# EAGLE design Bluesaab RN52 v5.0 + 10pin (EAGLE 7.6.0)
Removed DFU switch! D3 CANNOT be a Schottky diode; needs to be a signal diode. Might as well make all diodes the same... Added 2 bypass caps to RN52 power line. Switched to SN65HVD234 for higher temp (also has Enable pin which needs pulled high). Added 10 pin connector for the daughter board Amplifier. - OTHERWISE, THE LEFT 4 COLUMNS NEED JUMPERED.
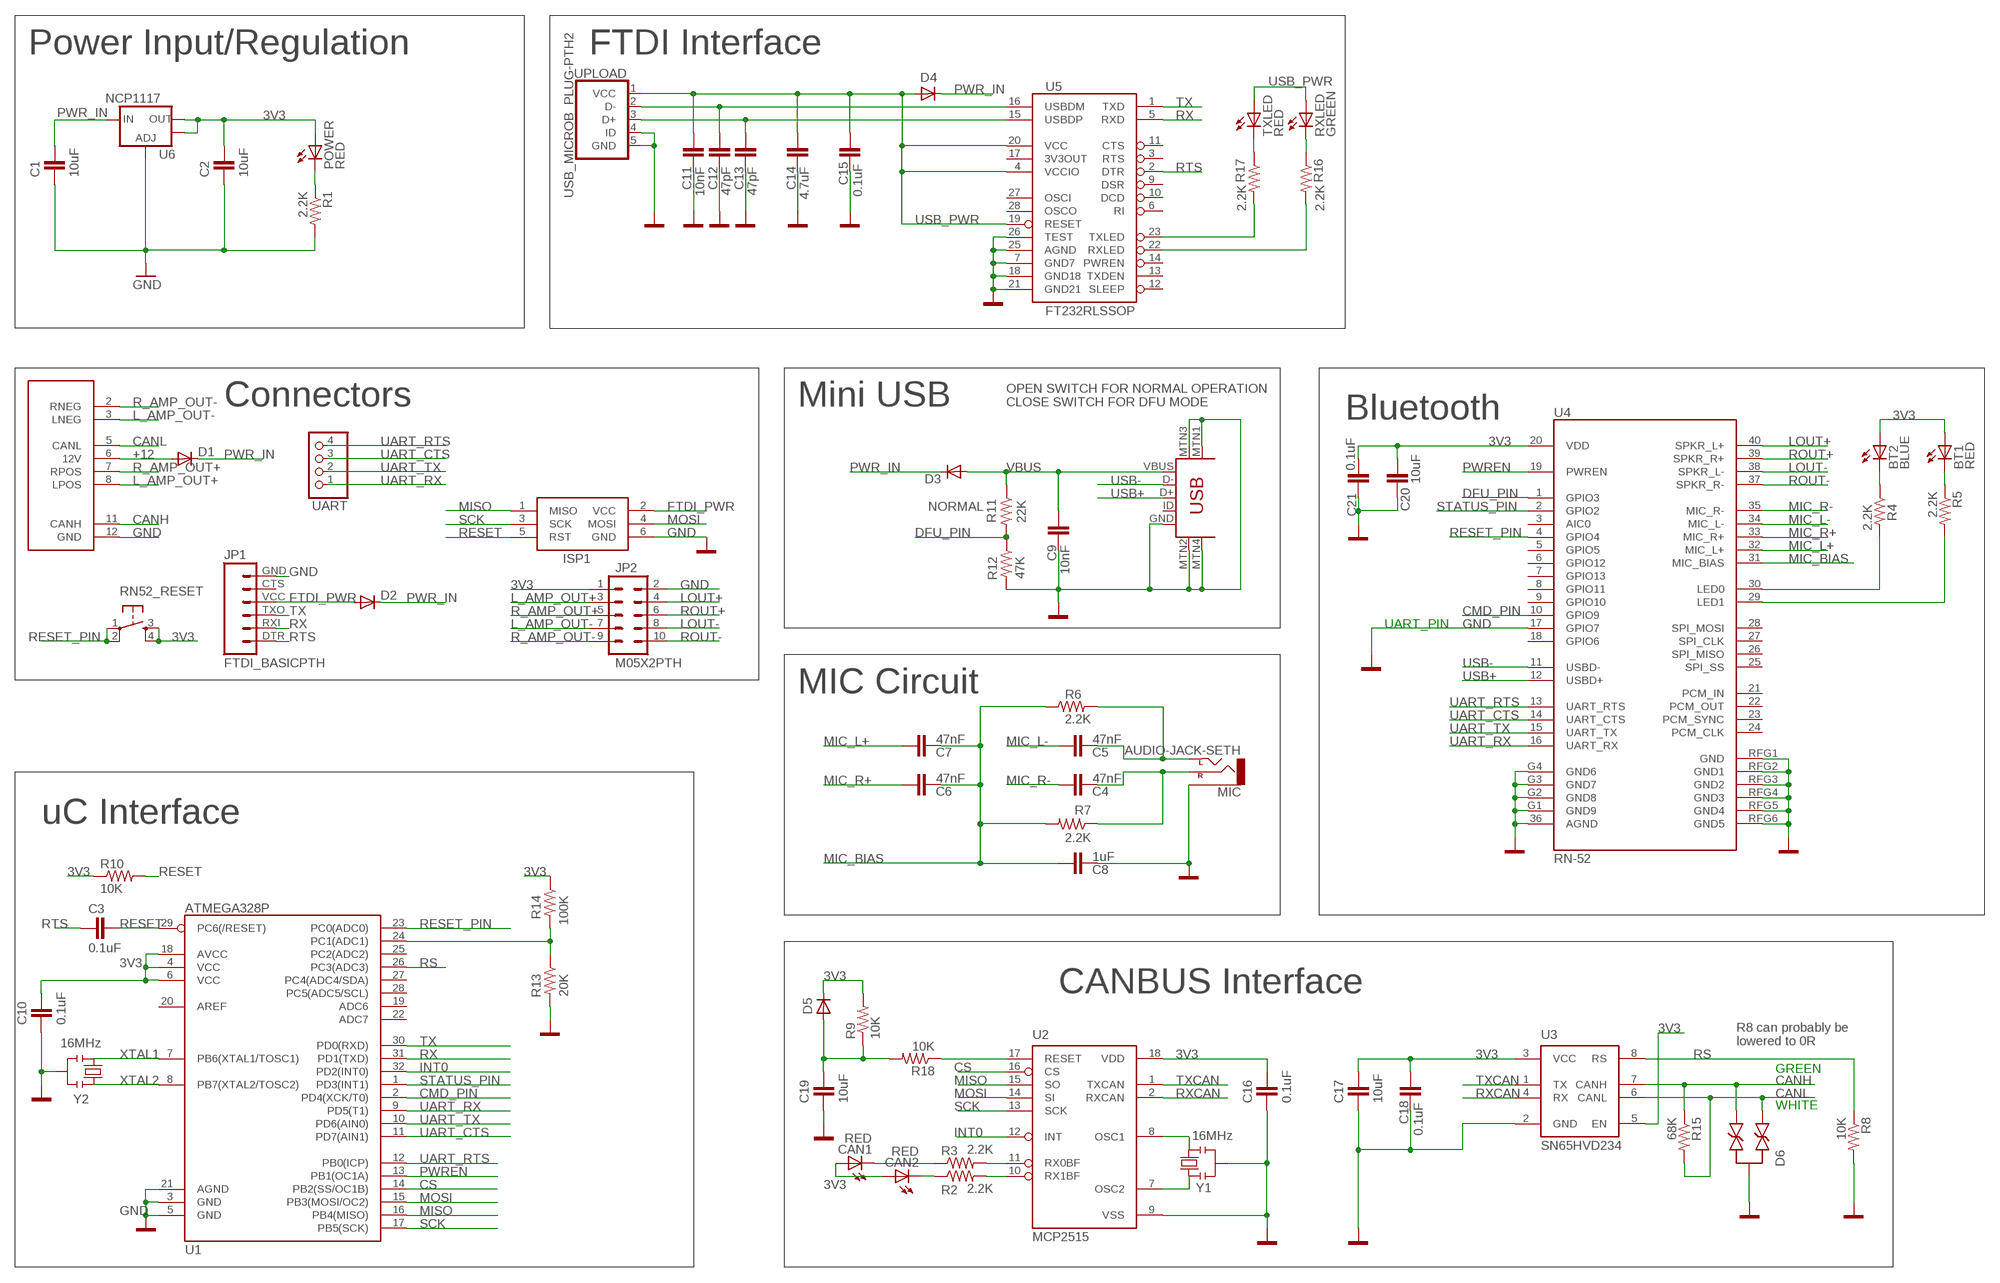
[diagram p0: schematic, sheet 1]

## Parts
BT1  RED  LEDSML1206  [SML1206]
BT2  BLUE  LEDSML1206  [SML1206]
C1  10uF  C-EUC0805K  [C0805K]
C2  10uF  C-EUC0805K  [C0805K]
C3  0.1uF  C-EUC0805K  [C0805K]
C4  47nF  C-EUC0805K  [C0805K]
C5  47nF  C-EUC0805K  [C0805K]
C6  47nF  C-EUC0805K  [C0805K]
C7  47nF  C-EUC0805K  [C0805K]
C8  1uF  C-EUC0805K  [C0805K]
C9  10nF  C-EUC0805K  [C0805K]
C10  0.1uF  C-EUC0805K  [C0805K]
C11  10nF  C-EUC0805K  [C0805K]
C12  47pF  C-EUC0805K  [C0805K]
C13  47pF  C-EUC0805K  [C0805K]
C14  4.7uF  C-EUC0805K  [C0805K]
C15  0.1uF  C-EUC0805K  [C0805K]
C16  0.1uF  C-EUC0805K  [C0805K]
C17  10uF  C-EUC0805K  [C0805K]
C18  0.1uF  C-EUC0805K  [C0805K]
C19  10uF  C-EUC0805K  [C0805K]
C20  10uF  C-EUC0805K  [C0805K]
C21  0.1uF  C-EUC0805K  [C0805K]
CAN1  RED  LEDSML1206  [SML1206]
CAN2  RED  LEDSML1206  [SML1206]
D1  DIODE-SCHOTTKY_  DIODE-SOD123  [SOD123]
D2  DIODE-SCHOTTKY_  DIODE-SOD123  [SOD123]
D3  DIODE-SCHOTTKY_  DIODE-SOD123  [SOD123]
D4  DIODE-SCHOTTKY_  DIODE-SOD123  [SOD123]
D5  DIODE-SCHOTTKY_  DIODE-SOD123  [SOD123]
D6  DIODE-ARRAY  [SOT23]
ISP1  AVRISP-6  [AVRISP]
JP1  FTDI_BASICPTH  [FTDI_BASIC]
JP2  M05X2PTH  [AVR_ICSP]
MIC  AUDIO-JACK-SETH  [AUDIO-JACK-3.5MM-SMD-SETH]
POWER  RED  LEDSML1206  [SML1206]
R1  2.2K  R-US_R0805  [R0805]
R2  2.2K  R-US_R0805  [R0805]
R3  2.2K  R-US_R0805  [R0805]
R4  2.2K  R-US_R0805  [R0805]
R5  2.2K  R-US_R0805  [R0805]
R6  2.2K  R-US_R0805  [R0805]
R7  2.2K  R-US_R0805  [R0805]
R8  10K  R-US_R0805  [R0805]
R9  10K  R-US_R0805  [R0805]
R10  10K  R-US_R0805  [R0805]
R11  22K  R-US_R0805  [R0805]
R12  47K  R-US_R0805  [R0805]
R13  20K  R-US_R0805  [R0805]
R14  100K  R-US_R0805  [R0805]
R15  68K  R-US_R0805  [R0805]
R16  2.2K  R-US_R0805  [R0805]
R17  2.2K  R-US_R0805  [R0805]
R18  10K  R-US_R0805  [R0805]
RN52_FIRMWARE  USB-MINIB-5PIN  [USB-MINIB]
RN52_RESET  TAC_SWITCH  [TACTILE_SWITCH_SMD_6MM]
RXLED  GREEN  LEDSML1206  [SML1206]
TXLED  RED  LEDSML1206  [SML1206]
U1  ATMEGA328P  ATMEGA328_SMT  [TQFP32-08]
U2  MCP2515  [SO18L]
U3  SN65HVD234  [SO8]
U4  RN-52  BLUETOOTH-RN-52  [RN-52]
U5  FT232RLSSOP  [SSOP28DB]
U6  NCP1117  V_REG_LM1117SOT223  [SOT223]
U$5  827229-1  [827229-1]
UART  PINHD-1X4  [1X04]
UPLOAD  USB_MICROB_PLUG-PTH2  [MICRO-B-TH]
Y1  16MHz  RESONATORSMD  [RESONATOR-SMD]
Y2  16MHz  RESONATORSMD  [RESONATOR-SMD]

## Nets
3V3: BT1.A BT2.A C2.2 C10.2 C16.2 C17.2 C18.1 C20.1 C21.2 CAN1.A CAN2.A D5.C JP2.1 POWER.A R9.2 R10.1 R14.1 RN52_RESET.3 RN52_RESET.4 U1.4(VCC) U1.6(VCC) U1.18(AVCC) U2.18(VDD) U3.3(VCC) U3.5(EN) U4.20(VDD) U6.2(OUT) U6.4(OUT)
+12 [12v]: D1.A U$5.6(12V)
CANH: D6.2 R15.1 U3.7(CANH) U$5.11(CANH)
CANL: D6.1 R15.2 U3.6(CANL) U$5.5(CANL)
CMD_PIN: U1.2(PD4(XCK/T0)) U4.10(GPIO9)
CS: U1.14(PB2(SS/OC1B)) U2.16(CS)
DFU_PIN: R11.2 R12.1 U4.1(GPIO3)
FTDI_PWR: D2.A ISP1.2(VCC) JP1.VCC
GND: C1.1 C2.1 C8.1 C9.1 C10.1 C11.1 C12.1 C13.1 C14.1 C15.2 C16.1 C17.1 C18.2 C19.1 C20.2 C21.1 D6.3 ISP1.6(GND) JP1.GND JP2.2 MIC.SLEEVE R1.2 R8.2 R12.2 R13.2 RN52_FIRMWARE.GND RN52_FIRMWARE.MTN1(MTN2) RN52_FIRMWARE.MTN2(MTN3) RN52_FIRMWARE.MTN3(MTN1) RN52_FIRMWARE.MTN4 U1.3(GND) U1.5(GND) U1.21(AGND) U2.9(VSS) U3.2(GND) U4.17(GPIO7) U4.36(AGND) U4.G1(GND9) U4.G2(GND8) U4.G3(GND7) U4.G4(GND6) U4.RFG1(GND) U4.RFG2(GND1) U4.RFG3(GND2) U4.RFG4(GND3) U4.RFG5(GND4) U4.RFG6(GND5) U5.7(GND7) U5.18(GND18) U5.21(GND21) U5.25(AGND) U5.26(TEST) U6.1(ADJ) U$5.12(GND) UPLOAD.4(ID) UPLOAD.5(GND) Y1.2 Y2.2
INT0: U1.32(PD2(INT0)) U2.12(INT)
L_AMP_OUT+: JP2.3 U$5.8(LPOS)
L_AMP_OUT-: JP2.7 U$5.3(LNEG)
LOUT+: JP2.4 U4.40(SPKR_L+)
LOUT-: JP2.8 U4.38(SPKR_L-)
MIC_BIAS: C6.1 C7.1 C8.2 R6.1 R7.2 U4.31(MIC_BIAS)
MIC_L+: C7.2 U4.32(MIC_L+)
MIC_L-: C5.1 U4.34(MIC_L-)
MIC_R+: C6.2 U4.33(MIC_R+)
MIC_R-: C4.1 U4.35(MIC_R-)
MISO: ISP1.1(MISO) U1.16(PB4(MISO)) U2.15(SO)
MOSI: ISP1.4(MOSI) U1.15(PB3(MOSI/OC2)) U2.14(SI)
N$1: R16.2 U5.22(RXLED)
N$4: U2.8(OSC1) Y1.3
N$5: U2.7(OSC2) Y1.1
N$6: BT2.C R4.1
N$7: BT1.C R5.1
N$8: R18.1 U2.17(RESET)
N$9: R13.1 R14.2 U1.24(PC1(ADC1))
N$10: R17.2 U5.23(TXLED)
N$12: R16.1 RXLED.C
N$13: CAN1.C R3.1
N$15: R17.1 TXLED.C
N$16: CAN2.C R2.1
N$17: POWER.C R1.1
N$18: R3.2 U2.11(RX0BF)
N$23: C4.2 MIC.RING(RIGHT) R7.1
N$25: C5.2 MIC.TIP(LEFT) R6.2
N$28: R5.2 U4.29(LED1)
N$29: R4.2 U4.30(LED0)
N$31: R2.2 U2.10(RX1BF)
N$35: C19.2 D5.A R9.1 R18.2
PWR_IN [12v]: C1.2 D1.C D2.C D3.C D4.C U6.3(IN)
PWREN: U1.13(PB1(OC1A)) U4.19(PWREN)
R_AMP_OUT+: JP2.5 U$5.7(RPOS)
R_AMP_OUT-: JP2.9 U$5.2(RNEG)
RESET: C3.2 ISP1.5(RST) R10.2 U1.29(PC6(/RESET))
RESET_PIN: RN52_RESET.1 RN52_RESET.2 U1.23(PC0(ADC0)) U4.4(GPIO4)
ROUT+: JP2.6 U4.39(SPKR_R+)
ROUT-: JP2.10 U4.37(SPKR_R-)
RS: R8.1 U1.26(PC3(ADC3)) U3.8(RS)
RTS: C3.1 JP1.DTR U5.2(DTR)
RX: JP1.RXI U1.31(PD1(TXD)) U5.5(RXD)
RXCAN: U2.2(RXCAN) U3.4(RX)
SCK: ISP1.3(SCK) U1.17(PB5(SCK)) U2.13(SCK)
STATUS_PIN: U1.1(PD3(INT1)) U4.2(GPIO2)
TX: JP1.TXO U1.30(PD0(RXD)) U5.1(TXD)
TXCAN: U2.1(TXCAN) U3.1(TX)
UART_CTS: U1.11(PD7(AIN1)) U4.14(UART_CTS) UART.3
UART_RTS: U1.12(PB0(ICP)) U4.13(UART_RTS) UART.4
UART_RX: U1.9(PD5(T1)) U4.16(UART_RX) UART.1
UART_TX: U1.10(PD6(AIN0)) U4.15(UART_TX) UART.2
USB+: RN52_FIRMWARE.D+ U4.12(USBD+)
USB-: RN52_FIRMWARE.D- U4.11(USBD-)
USB_PWR: C11.2 C14.2 C15.1 D4.A RXLED.A TXLED.A U5.4(VCCIO) U5.19(RESET) U5.20(VCC) UPLOAD.1(VCC)
USBDM: C12.2 U5.16(USBDM) UPLOAD.2(D-)
USBDP: C13.2 U5.15(USBDP) UPLOAD.3(D+)
VBUS: C9.2 D3.A R11.1 RN52_FIRMWARE.VBUS
XTAL1: U1.7(PB6(XTAL1/TOSC1)) Y2.1
XTAL2: U1.8(PB7(XTAL2/TOSC2)) Y2.3
Unconnected: JP1.CTS RN52_FIRMWARE.ID U1.19(ADC6) U1.20(AREF) U1.22(ADC7) U1.25(PC2(ADC2)) U1.27(PC4(ADC4/SDA)) U1.28(PC5(ADC5/SCL)) U4.3(AIC0) U4.5(GPIO5) U4.6(GPIO12) U4.7(GPIO13) U4.8(GPIO11) U4.9(GPIO10) U4.18(GPIO6) U4.21(PCM_IN) U4.22(PCM_OUT) U4.23(PCM_SYNC) U4.24(PCM_CLK) U4.25(SPI_SS) U4.26(SPI_MISO) U4.27(SPI_CLK) U4.28(SPI_MOSI) U5.3(RTS) U5.6(RI) U5.9(DSR) U5.10(DCD) U5.11(CTS) U5.12(SLEEP) U5.13(TXDEN) U5.14(PWREN) U5.17(3V3OUT) U5.27(OSCI) U5.28(OSCO)

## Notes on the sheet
- Power Input/Regulation | FTDI Interface
- Connectors | Mini USB
- OPEN SWITCH FOR NORMAL OPERATION
  CLOSE SWITCH FOR DFU MODE
- Bluetooth
- NORMAL
- UART_PIN
- MIC Circuit
- uC Interface
- CANBUS Interface
- R8 can probably be
  lowered to 0R
- GREEN
- WHITE

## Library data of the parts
BT1 BT2 CAN1 CAN2 POWER RXLED TXLED = led:LED: LED
C1-C21 = rcl:C-EU: CAPACITOR, European symbol
D1-D5 = diode_seth:DIODE-: DIODE
D6 = SparkFun-seth:DIODE-ARRAY: NUP2105L, TVS Diode Array
ISP1 = adafruit:AVRISP: AVR ISP HEADER Standard 6 pin header for AVR programming
JP1 = SparkFun-seth:FTDI_BASIC: FTDI Basic: 3.3V and 5V
JP2 = SparkFun-Connectors:M05X2: Header 5x2 Standard 10-pin dual row 0.1" header. Commonly used with AVR-ISP. Use with Spark Fun Electronics SKU: PRT-00778
MIC = SparkFun-Connectors:AUDIO-JACK-SETH
R1-R18 = rcl:R-US_: RESISTOR, American symbol
RN52_FIRMWARE = SparkFun-Connectors:USB-MINIB: Mini-USB "B" connector with 5th pin broken out. Created new symbol breaking out 5th "ID" pin in mini/micro USB connector spec. See: http://en.wikipedia.org/wiki/Mini_usb#Cables. Uses same footprint as 4-pin symbol. Also added pins to connect to mounting / shield pads if required (probably not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
RN52_RESET = SparkFun-seth:TAC_SWITCH: Momentary Switch Button commonly used for reset or general input. Spark Fun Electronics SKU : COM-00097
U1 = SparkFun-DigitalIC:ATMEGA328_SMT: 32-Pin Atmega328 part Commonly used on Arduino compatible boards Available in QFP and QFN packages TQFP is IC-09069 QFN is non-stock; PROD_ID: IC-09069
U2 = mcp2515-seth:MCP2515
U3 = ti-can-seth:SN65HVD234
U4 = SparkFun-RF:BLUETOOTH-RN-52
U5 = SparkFun-DigitalIC:FT232RL: USB UART FT232RL 4th Generation USB UART (USB <-> Serial) Controller. Spark Fun Electronics SKU : COM-00650 Production SKU IC-00870; PROD_ID: IC-00870
U6 = SparkFun:V_REG_LM1117: Voltage Regulator LM1117 Standard adjustable voltage regulator but in SMD form. Spark Fun Electronics SKU : COM-00595
U$5 = 827229-1:827229-1
UART = pinhead:PINHD-1X4: PIN HEADER
UPLOAD = SparkFun-Connectors-seth:USB_MICROB_PLUG: USB Micro-B Plug Comes in a variety of packages. Check out Hirose's ZX-x0 line: http://www.hirose.co.jp/cataloge_hp/e24200011.pdf
Y1 Y2 = SparkFun-seth:RESONATOR: Resonator Small SMD resonator. This is the itty bitty 10/20MHz resonators with built in caps. CSTCE10M0G55 and CSTCE20M0V53. Footprint has been reviewed closely but hasn't been tested yet.

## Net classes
0 default: width 0.254 mm
1 12v: width 0.5 mm

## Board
New PCB design, based on v4.4, NOW with 0805 resistors and caps. Adjusted layout to account for smaller parts.
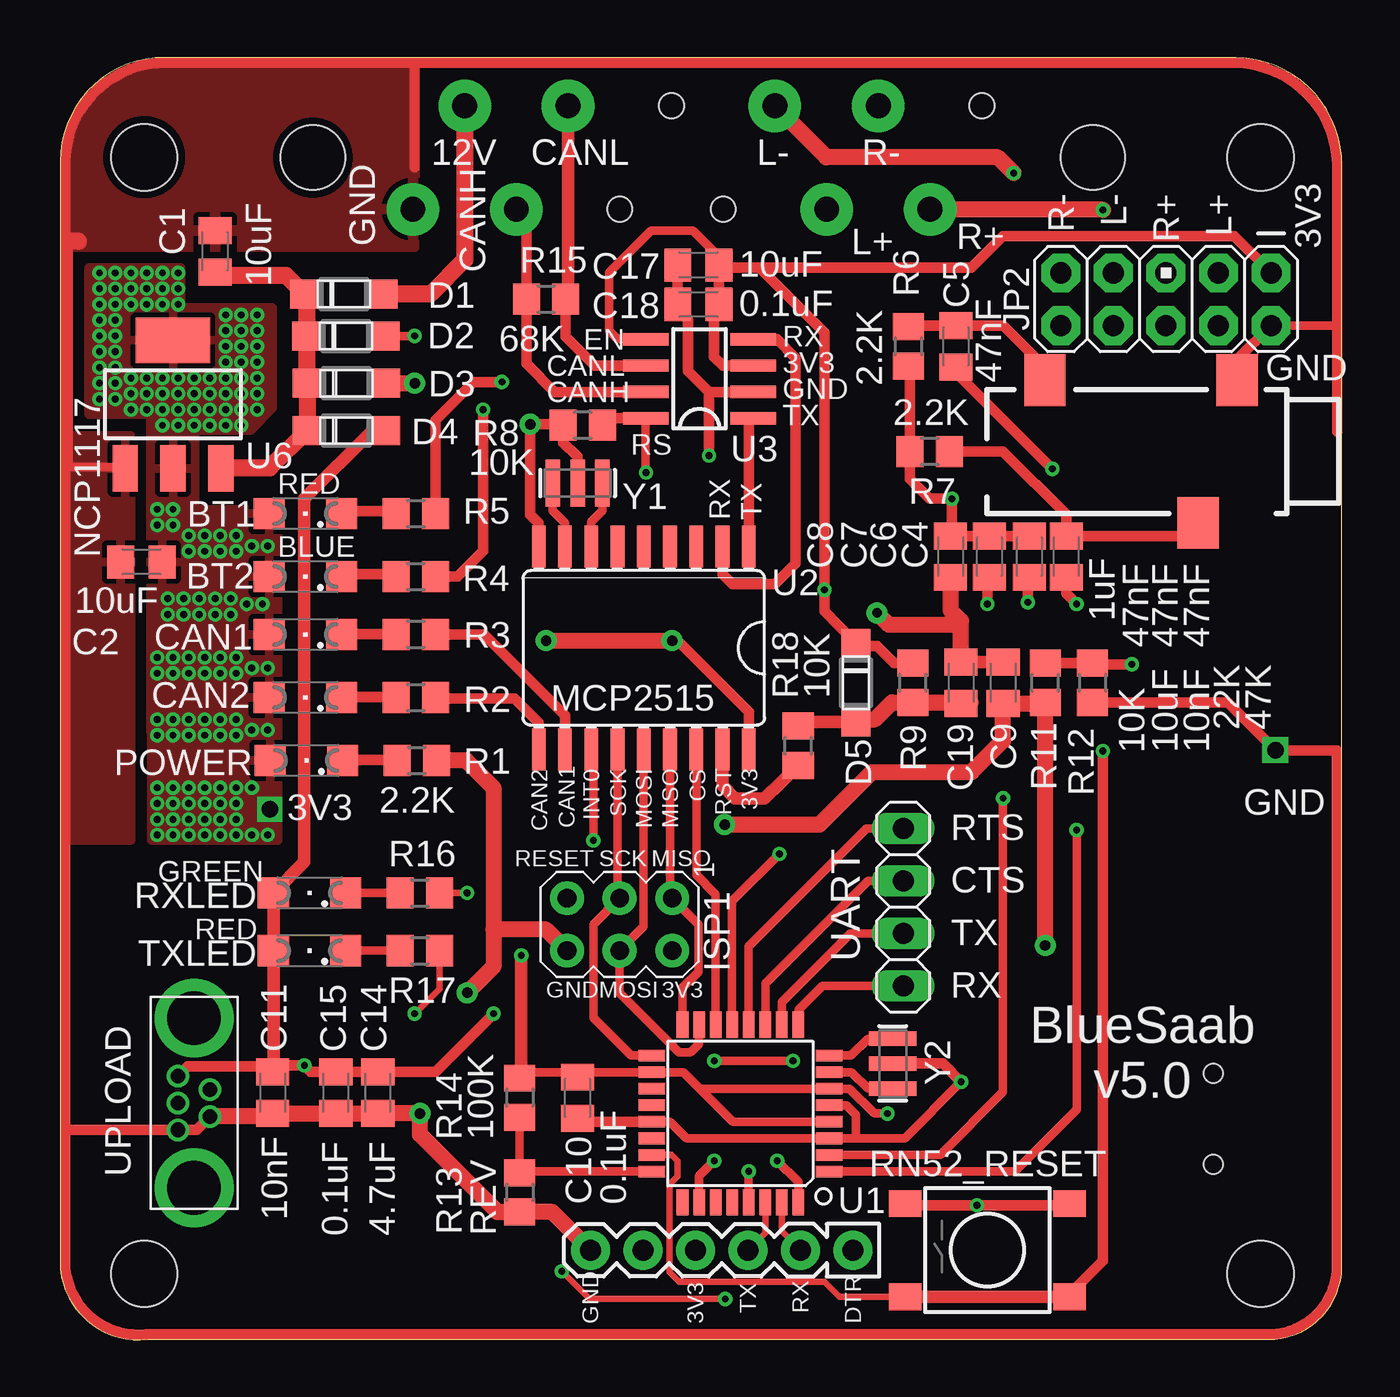
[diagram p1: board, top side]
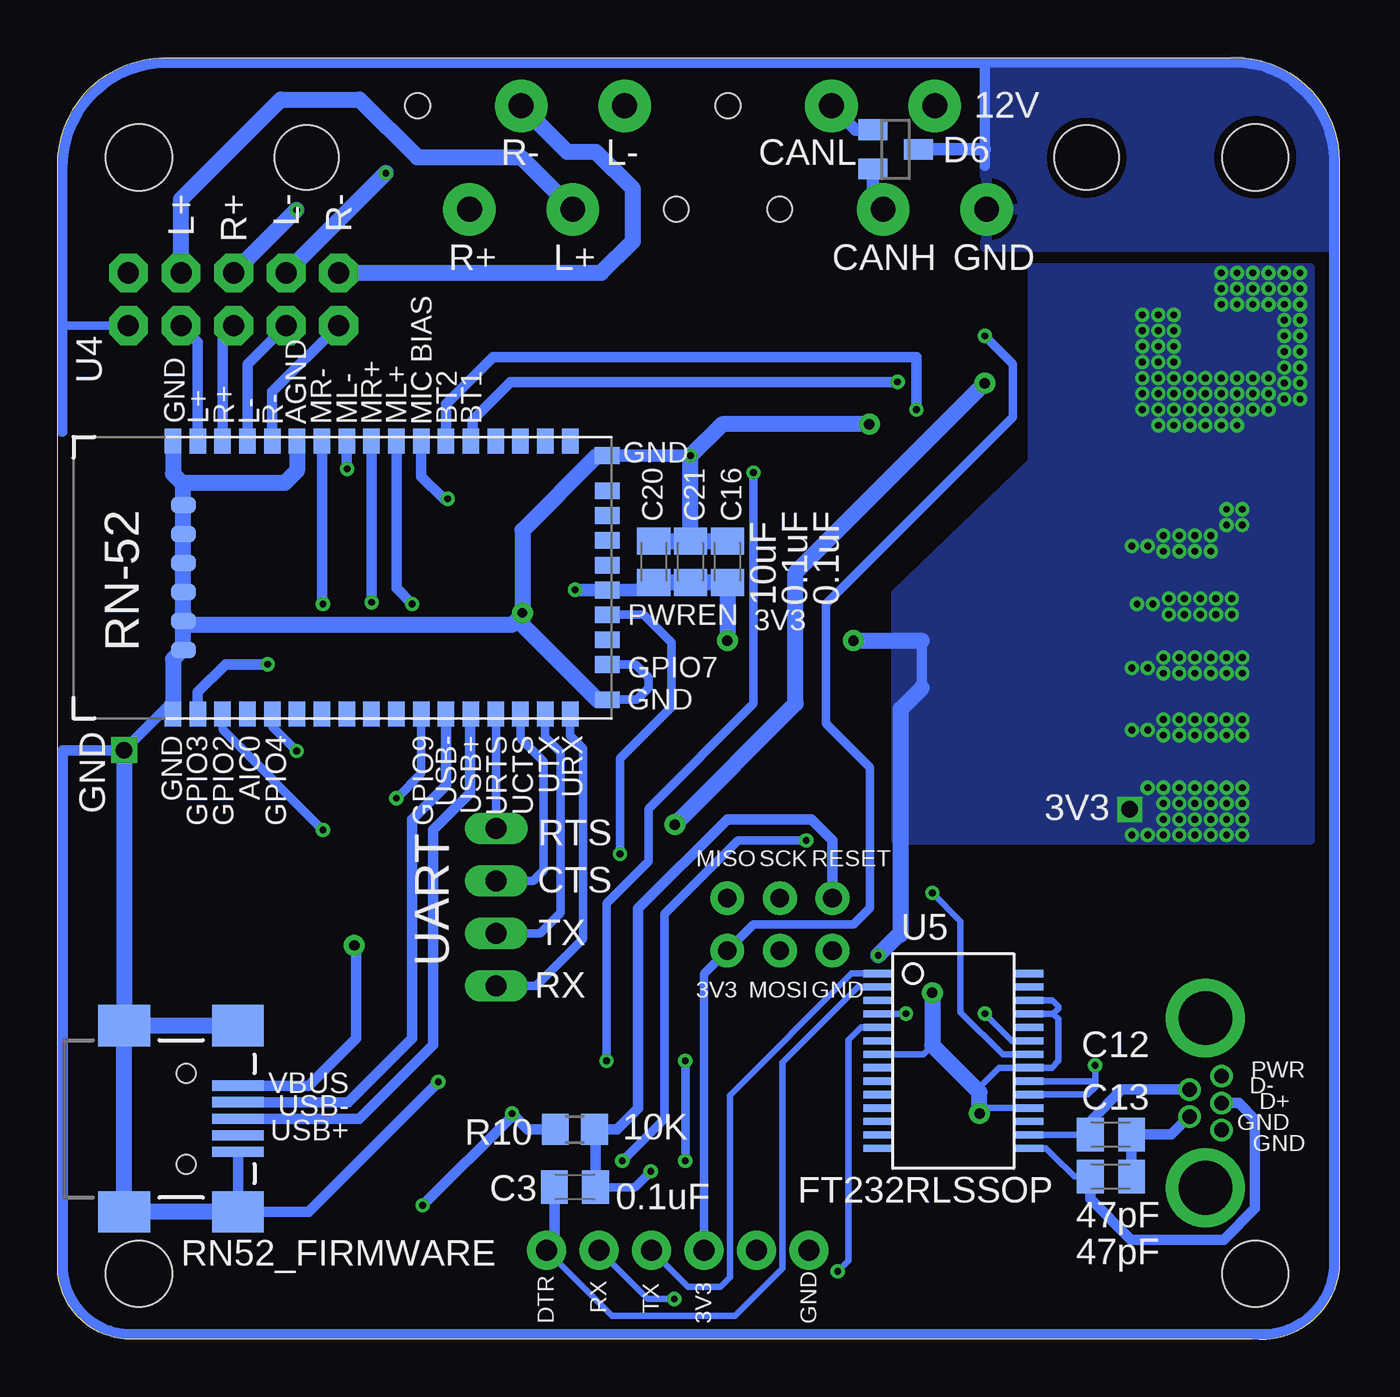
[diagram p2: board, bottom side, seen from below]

Size 61.98 x 62 mm. Coordinates in mm from the lower left corner, seen from the top.
Outline: 56.86,62 5.06,62 arc90 0,56.97 0,3.42 arc90 4.24,0.02 58.4,0.02 arc90 61.98,3.53 61.98,56.71 arc90 56.86,62
Copper layers (1*16): Top 0.0356mm / dielectric 1.5011mm / Bottom 0.0356mm
Design rules "OSHPark": minimum track width 6mil, minimum drill 13mil, track to track 6mil, track to pad 6mil, pad to pad 6mil, via to via 6mil, smd to smd 6mil, copper to edge 15mil, drill to drill 6mil, minimum pad ring 7mil, minimum via ring 7mil, stop-mask expansion 4mil, vias tented up to drill 0mil, thermal gap 10mil
Holes 3.2 mm at 4.06,57.17 58.04,57.17 58.04,3.2 4.06,3.2

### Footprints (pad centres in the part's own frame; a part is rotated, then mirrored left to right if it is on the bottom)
SML1206 = smd 1.5 x 1.5: A 1.75,0; C -1.75,0
C0805K = smd 1.3 x 1.6: 1 -1,0; 2 1,0
SOD123 = smd 1.4 x 1.4: A 1.9,0; C -1.9,0
SOT23 = smd 1 x 1.4: 1 -0.95,-1.1; 2 0.95,-1.1; 3 0,1.1
AVRISP = drill 0.9 pad 1.626: 1 -1.27,2.54; 2 1.27,2.54; 3 -1.27,0; 4 1.27,0; 5 -1.27,-2.54; 6 1.27,-2.54
FTDI_BASIC = drill 1.016 pad 1.88: CTS 10.16,0; DTR 0,0; GND 12.7,0; RXI 2.54,0; TXO 5.08,0; VCC 7.62,0
AVR_ICSP = drill 1.016 pad 1.88 octagon: 1 -1.27,5.08; 2 1.27,5.08; 3 -1.27,2.54; 4 1.27,2.54; 5 -1.27,0; 6 1.27,0; 7 -1.27,-2.54; 8 1.27,-2.54; 9 -1.27,-5.08; 10 1.27,-5.08
AUDIO-JACK-3.5MM-SMD-SETH = smd 2 x 2.5: RING 4.3,3.45; SLEEVE 2.4,-3.45; TIP 11.7,-3.45
R0805 = smd 1.3 x 1.5: 1 -0.95,0; 2 0.95,0
USB-MINIB = smd 2.5 x 0.5: D+ 2.5,0; D- 2.5,0.8; GND 2.5,-1.6; ID 2.5,-0.8; VBUS 2.5,1.6 | smd 2.5 x 2: MTN1 -3,4.5; MTN2 2.5,4.5; MTN3 -3,-4.5; MTN4 2.5,-4.5 | hole 0.9: 0,2.2; 0,-2.2
TACTILE_SWITCH_SMD_6MM = smd 1.55 x 1.3: 1 -3.975,2.25; 2 3.975,2.25; 3 -3.975,-2.25; 4 3.975,-2.25
TQFP32-08 = smd 1.27 x 0.559: 1 -4.293,2.8; 2 -4.293,2; 3 -4.293,1.2; 4 -4.293,0.4; 5 -4.293,-0.4; 6 -4.293,-1.2; 7 -4.293,-2; 8 -4.293,-2.8; 17 4.293,-2.8; 18 4.293,-2; 19 4.293,-1.2; 20 4.293,-0.4; 21 4.293,0.4; 22 4.293,1.2; 23 4.293,2; 24 4.293,2.8 | smd 0.559 x 1.27: 9 -2.8,-4.293; 10 -2,-4.293; 11 -1.2,-4.293; 12 -0.4,-4.293; 13 0.4,-4.293; 14 1.2,-4.293; 15 2,-4.293; 16 2.8,-4.293; 25 2.8,4.293; 26 2,4.293; 27 1.2,4.293; 28 0.4,4.293; 29 -0.4,4.293; 30 -1.2,4.293; 31 -2,4.293; 32 -2.8,4.293
SO18L = smd 0.66 x 2.032: 1 -5.08,-4.902; 2 -3.81,-4.902; 3 -2.54,-4.902; 4 -1.27,-4.902; 5 0,-4.902; 6 1.27,-4.902; 7 2.54,-4.902; 8 3.81,-4.902; 9 5.08,-4.902; 10 5.08,4.902; 11 3.81,4.902; 12 2.54,4.902; 13 1.27,4.902; 14 0,4.902; 15 -1.27,4.902; 16 -2.54,4.902; 17 -3.81,4.902; 18 -5.08,4.902
SO8 = smd 0.6 x 2.2: 1 -1.905,-2.6; 2 -0.635,-2.6; 3 0.635,-2.6; 4 1.905,-2.6; 5 1.905,2.6; 6 0.635,2.6; 7 -0.635,2.6; 8 -1.905,2.6
RN-52 = smd 1.2 x 0.8: 1 -6.6,8.33; 2 -6.6,7.13; 3 -6.6,5.93; 4 -6.6,4.73; 5 -6.6,3.53; 6 -6.6,2.33; 7 -6.6,1.13; 8 -6.6,-0.07; 9 -6.6,-1.27; 10 -6.6,-2.47; 11 -6.6,-3.67; 12 -6.6,-4.87; 13 -6.6,-6.07; 14 -6.6,-7.27; 15 -6.6,-8.47; 16 -6.6,-9.67; 25 6.6,-9.67; 26 6.6,-8.47; 27 6.6,-7.27; 28 6.6,-6.07; 29 6.6,-4.87; 30 6.6,-3.67; 31 6.6,-2.47; 32 6.6,-1.27; 33 6.6,-0.07; 34 6.6,1.13; 35 6.6,2.33; 36 6.6,3.53; 37 6.6,4.73; 38 6.6,5.93; 39 6.6,7.13; 40 6.6,8.33; G1 -6.6,9.53; G4 6.6,9.53 | smd 0.8 x 1.2: 17 -4.2,-11.47; 18 -3,-11.47; 19 -1.8,-11.47; 20 -0.6,-11.47; 21 0.6,-11.47; 22 1.8,-11.47; 23 3,-11.47; 24 4.2,-11.47; G2 -5.9,-11.47; G3 5.9,-11.46; RFG1 -3.5,9.03; RFG2 -2.1,9.03; RFG3 -0.7,9.03; RFG4 0.7,9.03; RFG5 2.1,9.03; RFG6 3.5,9.03
SSOP28DB = smd 0.348 x 1.397: 1 -4.225,-3.656; 2 -3.575,-3.656; 3 -2.925,-3.656; 4 -2.275,-3.656; 5 -1.625,-3.656; 6 -0.975,-3.656; 7 -0.325,-3.656; 8 0.325,-3.656; 9 0.975,-3.656; 10 1.625,-3.656; 11 2.275,-3.656; 12 2.925,-3.656; 13 3.575,-3.656; 14 4.225,-3.656; 15 4.225,3.656; 16 3.575,3.656; 17 2.925,3.656; 18 2.275,3.656; 19 1.625,3.656; 20 0.975,3.656; 21 0.325,3.656; 22 -0.325,3.656; 23 -0.975,3.656; 24 -1.625,3.656; 25 -2.275,3.656; 26 -2.925,3.656; 27 -3.575,3.656; 28 -4.225,3.656
SOT223 = smd 1.219 x 2.235: 1 -2.311,-3.099; 2 0,-3.099; 3 2.311,-3.099 | smd 3.6 x 2.2: 4 0,3.099
827229-1 = drill 1.2 pad 2.54: 2 2.96,-9.495; 3 2.96,-4.495; 5 2.96,5.505; 6 2.96,10.505; 7 -2.04,-11.995; 8 -2.04,-6.995; 11 -2.04,8.005; 12 -2.04,13.005 | hole 3.1: 0.46,17.84; 0.46,-19.86 | hole 1.2: -2.04,3.005; 2.96,-14.495; -2.04,-1.995; 2.96,0.505
1X04 = drill 1.016 long: 1 -3.81,0; 2 -1.27,0; 3 1.27,0; 4 3.81,0
MICRO-B-TH = drill 0.711 pad 1.092: 1 -1.3,-0.775; 2 -0.65,0.775; 3 0,-0.775; 4 0.65,0.775; 5 1.3,-0.775 | drill 2.591 pad 3.81: P$1 -4.1,0; P$2 4.1,0
RESONATOR-SMD = smd 0.7 x 2.286: 1 -1.2,0; 2 0,0; 3 1.2,0

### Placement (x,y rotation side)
BT1  11.86,39.95 180 top
BT2  11.86,36.9 180 top
C1  7.49,52.63 270 top
C2  3.94,37.61 0 top
C3  36.96,7.39 0 bottom
C4  48.64,37.87 90 top
C5  43.31,48.03 90 top
C6  46.86,37.87 270 top
C7  44.93,37.87 270 top
C8  43.05,37.87 90 top
C9  45.59,31.77 270 top
C10  25.02,11.71 90 top
C11  10.29,11.96 90 top
C12  11.05,9.93 180 bottom
C13  11.05,7.9 180 bottom
C14  15.37,11.96 90 top
C15  13.33,11.96 270 top
C16  29.59,37.61 270 bottom
C17  30.86,51.97 0 top
C18  30.86,50.06 180 top
C19  43.56,31.77 270 top
C20  33.15,37.61 90 bottom
C21  31.37,37.61 270 bottom
CAN1  11.86,34.11 180 top
CAN2  11.86,31.06 180 top
D1  13.72,50.57 0 top
D2  13.82,48.54 0 top
D3  13.84,46.25 0 top
D4  13.84,43.96 0 top
D5  38.48,31.77 270 top
D6  21.46,57.55 270 bottom
ISP1  27.05,20.09 270 top
JP1  38.34,4.34 180 top
JP2  53.47,50.31 270 top
MIC  59.31,42.95 180 top
POWER  11.91,28.01 180 top
R1  17.25,28.01 0 top
R2  17.2,31.06 0 top
R3  17.2,34.11 0 top
R4  17.2,36.9 0 top
R5  17.2,39.95 0 top
R6  41.02,48.03 90 top
R7  42.04,42.95 180 top
R8  25.27,44.22 180 top
R9  41.23,31.77 90 top
R10  36.96,10.18 0 bottom
R11  47.62,31.77 90 top
R12  49.91,31.77 270 top
R13  22.23,7.13 270 top
R14  22.23,11.71 270 top
R15  23.5,50.31 0 top
R16  17.4,21.61 0 top
R17  17.4,18.82 0 top
R18  35.69,28.72 90 top
RN52_FIRMWARE  55.75,10.69 0 bottom
RN52_RESET  44.83,4.34 180 top
RXLED  12.06,21.61 180 top
TXLED  12.06,18.82 180 top
U1  32.89,10.94 180 top
U2  28.22,33.45 180 top
U3  30.92,46.47 90 top
U4  46.86,36.85 90 bottom
U5  18.67,13.48 270 bottom
U6  5.46,45.23 0 top
U$5  30.07,56.7 90 top
UART  40.77,20.93 90 top
UPLOAD  6.48,11.45 270 top
Y1  25.02,41.42 180 top
Y2  40.26,13.36 90 top

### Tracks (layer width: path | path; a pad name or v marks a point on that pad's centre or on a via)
3V3  (via drill 0.33, 0.5 pad 1.02, 0.8)
  Top 0.305: v22.3,18.6 22.33,18.56 v22.3,18.59 | 10.13,27.99 POWER.A
  Top 0.406: R14.1 22.3,12.94 24.77,12.94 | 24.77,12.94 U1.18 30.13,12.94 30.93,12.14 | v40,10.94 39.37,10.94 38.17,12.14 U1.6 30.93,12.14 | C10.2 25.02,12.69 24.77,12.94 | U1.4 32.53,10.54 30.93,12.14 | U3.5 26.96,48.37 26.54,48.79 26.54,51.58 28.58,53.62 30.61,53.62 31.86,52.36 C17.2
  Top 0.5: 10.21,31.09 CAN2.A 10.21,30.93 | 10.21,33.98 CAN1.A 10.21,34.29 | 10.21,36.88 BT2.A | 10.21,37.03 BT2.A | 10.24,39.85 BT1.A 9.93,39.85 | 10.24,37.26 BT2.A | 10.21,28.06 POWER.A | U2.18 | 36.96,47.64 36.96,48.69 33.81,51.84 33.4,51.84 31.98,51.84 | U1.18 | U3.3 32.04,47.1 31.62,47.52 31.62,49.83 C18.1 C17.2 | D5.C 38.6,33.55 39.5,33.55
  Top 0.508: 36.96,47.64 v36.96,36.27 36.96,35.23 38.45,33.7 arc-90 D5.C | 39.5,33.55 40.32,32.72 R9.2 | 31.98,51.84 C17.2 | v29.59,33.8 29.85,33.8 33.3,30.35 U2.18 | RN52_RESET.3 arc-90 49.22,6.5 v44.32,6.5 41.45,6.5 RN52_RESET.4 | JP2.1 56.77,53.36 45.59,53.36 44.07,51.84 33.4,51.84
  Top 0.61: CAN1.A 10.06,34.06 | 22.3,12.94 v22.3,18.6
  Top 0.762: 10.24,39.85 10.11,39.73 | 10.21,36.88 10.11,36.78 | 10.21,33.98 10.11,33.88 | 10.21,30.93 10.16,30.89 | 10.07,39.91 arc90 BT1.A | v23.5,33.8 v29.59,33.8
  Top 0.813: 5.41,48.28 U6.4
  Bottom 0.305: 21.21,19.58 21.31,19.58
  Bottom 0.5: 35.56,36.28 U4.20 | v44.32,6.5 40,10.82 v40,10.94
  Bottom 0.508: R10.1 39.24,10.18 v40,10.94 | 20.19,33.8 20.19,31.52
  Bottom 0.61: v36.96,36.27 36.94,36.25 U4.20 34.02,36.25 C20.1
  Bottom 0.762: 21.21,19.58 21.21,30.5 20.19,31.52 | 21.31,19.58 v22.3,18.59 | v23.5,33.8 20.19,33.8 | v29.59,33.8 C16.2 C21.2 C20.1
  other vias: 10.13,25.65 1.91,51.58 2.67,47.77 1.91,50.06 4.19,44.98 5.71,45.74 8.76,47.27 8.76,45.74 2.67,50.82 1.91,48.54 1.91,47.01 2.67,46.25 5.71,44.98 8,44.22 9.52,46.5 9.52,49.55 4.95,51.58 2.67,49.3 4.19,45.74 9.52,44.98 9.52,48.03 3.43,51.58 4.19,50.82 3.43,50.06 4.95,50.06 8,49.55 4.95,44.22 6.48,44.22 8.76,44.22 7.24,46.5 5.46,40.15 4.7,29.99 6.99,29.99 6.73,35.84 5.46,29.23 4.7,40.15 5.46,25.93 2.67,51.58 1.91,50.82 4.19,51.58 3.43,50.82 1.91,49.3 2.67,48.54 1.91,47.77 1.91,46.25 2.67,50.06 2.67,47.01 3.43,45.74 4.95,44.98 4.95,45.74 6.48,44.98 5.71,44.22 7.24,44.22 7.24,45.74 8.76,44.98 9.52,45.74 8.76,46.5 8,47.27 9.52,47.27 8,48.03 8.76,49.55 8.76,48.03 4.19,50.06 4.95,50.82 3.43,46.5 4.95,46.5 5.71,46.5 3.43,44.98 4.19,46.5 6.48,46.5 6.48,45.74 7.24,44.98 8,44.98 8,45.74 8,46.5 8,48.79 8.76,48.79 9.52,48.79 5.71,51.58 5.71,50.82 5.71,50.06 2.67,45.49 1.91,45.49 4.7,39.39 4.7,29.23 6.22,29.99 5.46,26.69 5.46,25.17 6.22,24.41 6.99,24.41 7.75,24.41 8.51,24.41 9.27,24.41 10.03,24.41 4.7,26.69 4.7,25.93 4.7,25.17 4.7,24.41 5.46,24.41 5.46,29.99 6.22,29.23 6.99,29.23 6.22,26.69 6.99,26.69 7.75,26.69 8.51,26.69 9.27,26.69 6.22,25.93 6.99,25.93 7.75,25.93 8.51,25.93 6.22,25.17 6.99,25.17 7.75,25.17 8.51,25.17 5.46,39.39 6.22,38.88 6.22,38.12 6.99,38.12 6.99,38.88 7.75,38.88 7.75,38.12 8.51,38.12 8.51,38.88 9.27,38.38 10.03,38.38 5.21,35.07 5.21,35.84 5.97,35.07 6.73,35.07 5.97,35.84 7.49,35.84 8.25,35.84 7.49,35.07 8.25,35.07 9.02,35.58 9.78,35.58 7.75,29.99 8.51,29.99 7.75,29.23 8.51,29.23 9.27,29.49 10.03,29.49 4.7,32.99 6.99,32.99 5.46,32.23 4.7,32.23 6.22,32.99 5.46,32.99 6.22,32.23 6.99,32.23 7.75,32.99 8.51,32.99 7.75,32.23 8.51,32.23 9.27,32.48 10.03,32.48
  pour Top: 1.4,51.84 1.4,44.73 4.37,44.73 4.39,24.15 10.54,24.15 10.54,40.15 6.53,40.15 6.53,43.96 9.21,43.96 10.29,45.04 10.29,49.91 5.87,49.91 5.87,51.84
  pour Bottom: 1.4,51.84 1.4,24.15 21.46,24.15 21.46,36.09 14.86,42.44 14.86,51.84
+12
  Top 0.813: U$5.6 19.56,52.22 17.91,50.57 D1.A
CANH
  Top 0.508: U$5.11 22.55,54.18 R15.1 22.55,47.2 23.91,45.83 U3.7
  Top 0.61: U$5.11
  Bottom 0.61: D6.2 22.56,55.16 U$5.11
CANL
  Top 0.508: U3.6 25.84,47.1 24.45,48.5 R15.2
  Top 0.61: R15.2 24.56,50.67 U$5.5
  Bottom 0.61: D6.1 23.4,58.5 U$5.5
CMD_PIN  (via drill 0.33)
  Top 0.406: v45.59,26.18 45.59,11.98 42.56,8.94 U1.2
  Bottom 0.406: U4.10 44.39,27.38 v45.59,26.18
  Bottom 0.5: 44.33,30.26 U4.10
CS
  Top 0.406: U2.16 30.76,22.48 31.69,21.54 U1.14
DFU_PIN  (via drill 0.33)
  Top 0.508: R11.2 R12.1 arc90 49.97,32.66 v51.82,32.66
  Bottom 0.5: 55.19,30.81 U4.1
  Bottom 0.508: 55.19,30.81 55.19,31.32 53.85,32.66 v51.82,32.66
FTDI_PWR  (via drill 0.33)
  Top 0.406: v17.14,48.54 D2.A
  Bottom 0.406: v17.14,48.54 15.79,47.19 15.79,44.6 24.3,36.09 24.82,35.58 24.82,29.79 22.71,27.68 22.71,20.87 23.5,20.09 28.32,20.09 ISP1.2 30.72,17.69 JP1.VCC
GND  (via drill 0.33, 0.46 pad 1.02, 0.5 pad 1.02, 0.8 pad 1.27)
  Top 0.406: 37.26,9.67 U1.3 | U1.21 29.48,10.54 30.28,9.74 U1.3 | 0.41,53.14 0.38,53.11 | 0.38,42.19 3.1,42.19 U6.1 | U1.3 38.41,9.74 | 38.41,9.74 38.48,9.81 38.48,10.87 38.01,11.34 U1.5 | 38.41,9.74 40.84,9.74 v43.56,12.47 | JP2.2 61.75,49.04 | 3.68,10.15 3.68,10.18
  Top 0.5: 18.42,28.03 R1.2 | Y2.2 42.67,13.36 v43.56,12.47 | UPLOAD.5 3.68,10.15 0.25,10.15 0.25,9.93 | 58.75,28.5 61.72,28.5 | 0.38,53.11 0.38,42.19 | C10.1 25.1,10.54 U1.21 | C18.2 C17.1 | 31.37,45.83 30.35,46.85 30.35,49.3 | 31.37,45.83 v31.37,42.75 | U3.2 31.37,45.83
  Top 0.508: 61.72,28.5 61.72,3.68 arc-90 58.55,0.28 4.17,0.28 arc-90 0.25,3.43 0.25,9.93 0.25,56.92 arc-90 5.11,61.74 17.14,61.74 | 17.14,61.74 17.14,56.69 | 17.14,61.74 56.52,61.74 arc-90 61.75,56.87 61.75,49.04 61.75,43.91 | UPLOAD.5 6.6,10.15 UPLOAD.4 | 30.35,49.3 29.86,49.79 C18.2 | Y1.2 25.02,42.69 24.32,43.39 R8.2 arc90 24.27,44.27 v22.73,44.27 22.73,39.9 23.14,39.49 U2.9 | R12.2 56.45,30.82 v58.75,28.52 | MIC.SLEEVE 56.91,47.41 JP2.2
  Top 0.61: C19.1 C9.1 | 24.51,44.15 arc-90 R8.2
  Top 0.762: 20.96,19.83 20.96,26.69 19.63,28.01 R1.2 | 20.96,19.83 20.96,18.06 v19.69,16.79 | ISP1.6 23.5,19.83 20.96,19.83 | UPLOAD.4 8.76,10.82 10.14,10.82 C11.1 C15.2 C14.1 17.14,10.96 v17.4,10.94 17.4,9.93 21.14,6.18 R13.2 23.8,6.18 JP1.GND | C19.1 43.56,34.76 | C8.1 43.05,35.27 43.56,34.76 | 43.56,34.76 43.37,34.57 40.08,34.57 v39.5,35.15
  Top 0.813: 0.41,53.14 0.86,53.14 0.89,53.11
  Bottom 0.305: U5.26 13.88,16.41 13.59,16.12 13.59,16.01 13.84,15.76 U5.25 15,15.77 13.84,15.77 13.59,15.52 13.59,13.48 13.91,13.16 U5.21 16.45,13.16 17.53,12.09 | U5.18 17.14,11.21 v17.4,10.94 | U5.7 20.12,13.81 19.69,14.25
  Bottom 0.406: U4.G2 33.97,30.95 33.4,31.52 33.4,32.03 34.03,32.65 U4.17 | JP2.2 61.75,49.04
  Bottom 0.5: 56.24,30.09 U4.G1 | U4.RFG1 55.89,33.41 | 61.72,28.5 58.75,28.5
  Bottom 0.508: RN52_FIRMWARE.GND RN52_FIRMWARE.MTN4 49.84,6.19 v43.56,12.47 | 35.43,30.91 U4.G2 | 17.14,61.74 5.18,61.77 arc90 0.25,57.07 0.25,3.45 arc90 4.04,0.28 58.55,0.28 arc90 61.72,3.71 61.72,28.5 | 17.14,61.74 17.14,57.55 17.14,56.78 | 56.52,61.74 56.77,61.74 arc-90 61.75,56.61 | 61.75,56.61 61.75,56.87 arc90 56.52,61.74 | 61.75,56.61 61.75,49.04 61.75,43.91 | 17.14,61.74 56.52,61.74 | C13.1 C12.1 8.13,9.93 UPLOAD.4 | U4.G1 56.39,30.69 56.26,30.82 56.45,30.82 v58.75,28.52
  Bottom 0.61: D6.3 17.14,57.55 | v31.37,42.75 U4.G3 35.88,42.75
  Bottom 0.762: v58.75,28.52 58.75,28.5 RN52_FIRMWARE.MTN1 | RN52_FIRMWARE.MTN2 RN52_FIRMWARE.MTN1 | RN52_FIRMWARE.MTN1 RN52_FIRMWARE.MTN3 RN52_FIRMWARE.MTN4 | v39.5,35.15 39.5,35.07 40,34.57 55.75,34.57 55.89,35.15 | 55.89,35.15 U4.RFG2 55.89,33.41 56.39,32.91 U4.G1 | U4.G4 56.39,41.87 55.95,41.42 55.75,41.42 | U4.36 50.39,42.02 50.98,41.42 55.75,41.42 | U4.G2 35.88,30.95 39.5,34.57 v39.5,35.15 | 55.89,35.15 U4.RFG3 U4.RFG4 U4.RFG5 U4.RFG6 55.89,41.28 55.75,41.42 | 35.88,42.75 39.5,39.14 v39.5,35.15 | v19.69,16.79 19.69,14.25 17.53,12.09 17.4,11.96 v17.4,10.94 | v22.73,44.27 29.84,44.27 v31.37,42.75 C21.1 | C20.2 C21.1 | C21.1 C16.1
  pour Top: 17.14,52.85 17.14,61.74 5.46,61.74 arc90 0.25,56.92 0.25,52.85
  pour Bottom: 17.14,52.85 17.14,61.74 5.46,61.74 arc90 0.25,56.92 0.25,52.85
  pour Top: 0.25,43.71 3.43,43.71 3.43,24.15 0.25,24.15
INT0  (via drill 0.33)
  Top 0.406: U1.32 35.69,7.64 v34.67,8.66 | v25.78,24.15 25.78,28.45 U2.12
  Bottom 0.406: v34.67,8.66 32.64,10.69 32.64,20.6 29.08,24.15 v25.78,24.15
L_AMP_OUT+
  Bottom 0.762: JP2.3 56.01,55.14 51.18,59.97 47.37,59.97 44.58,57.17 39.57,57.17 U$5.8
L_AMP_OUT-  (via drill 0.33)
  Top 0.762: v46.1,56.41 45.34,57.17 37.05,57.17 U$5.3
  Bottom 0.762: JP2.7 v46.1,56.41
LOUT+
  Bottom 0.508: U4.40 55.19,48.23 JP2.4
LOUT-
  Bottom 0.508: U4.38 52.79,47.18 JP2.8
MIC_BIAS  (via drill 0.33)
  Top 0.5: C7.1 C6.1
  Top 0.508: 43.07,38.87 C7.1 | 42.67,38.87 C8.2 43.07,38.87 | R6.1 41.09,47.01 R7.2 41.09,41.61 42.04,40.66 v43.12,40.66 43.12,39.07 43.07,38.87
  Bottom 0.508: v43.12,40.66 43.31,40.66 44.39,41.75 U4.31
MIC_L+  (via drill 0.33)
  Top 0.508: C7.2 44.83,36.85 v44.83,35.58
  Bottom 0.5: U4.32 45.59,36.34 v44.83,35.58
MIC_L-  (via drill 0.33)
  Top 0.508: v47.98,42.11 47.88,42.19 43.31,46.76 C5.1
  Bottom 0.508: v47.98,42.11 47.99,42.07 U4.34
MIC_R+  (via drill 0.33)
  Top 0.508: C6.2 arc90 46.79,36.79 v46.79,35.66
  Bottom 0.5: U4.33 v46.79,35.66
MIC_R-  (via drill 0.33)
  Top 0.508: C4.1 48.64,36.09 v49.15,35.58
  Bottom 0.508: v49.15,35.58 49.19,35.63 U4.35
MISO
  Top 0.406: U2.15 29.49,21.46 ISP1.1 30.86,20.09 30.86,17.8 30.09,17.03 U1.16
MOSI
  Top 0.406: U2.14 28.22,19.99 ISP1.4 27.05,16.79 29.93,13.91 30.48,13.91 30.89,14.32 U1.15
N$1  (via drill 0.33)
  Top 0.305: v19.69,21.61 R16.2
  Bottom 0.305: U5.22 16.28,13.81 18.31,15.84 18.31,20.24 v19.69,21.61
N$4
  Top 0.406: Y1.3 23.82,40.08 24.41,39.49 U2.8
N$5
  Top 0.406: U2.7 25.68,39.54 26.22,40.08 Y1.1
N$6
  Top 0.5: BT2.C 13.72,37.03 15.7,37.03 R4.1
N$7
  Top 0.5: BT1.C 13.72,40.08 15.7,40.08 R5.1
N$8
  Top 0.61: R18.1 34.06,26.18 32.64,26.18 32.03,26.79 U2.17
N$9
  Top 0.305: R13.1 22.29,8.15 22.73,8.15
  Top 0.406: R14.2 R13.1 | U1.24 27.57,8.14 22.73,8.15
N$10  (via drill 0.33)
  Top 0.305: R17.2 18.35,16.97 v17.14,15.77
  Bottom 0.305: U5.23 15.83,14.46 v17.14,15.77
N$12
  Top 0.406: RXLED.C R16.1
N$13
  Top 0.5: CAN1.C 13.72,34.13 15.7,34.13 R3.1
N$15
  Top 0.406: TXLED.C R17.1
N$16
  Top 0.5: CAN2.C 13.72,31.09 15.7,31.09 R2.1
N$17
  Top 0.5: POWER.C 13.72,28.04 15.7,28.04 R1.1
N$18
  Top 0.5: R3.2 20.49,34.11 24.41,30.19 U2.11
N$23
  Top 0.508: R7.1 45.59,42.95 48.64,39.9 C4.2 54.38,38.87 arc90 MIC.RING
N$25
  Top 0.508: R6.2 41.07,49.03 C5.2 45.61,49.03 47.12,47.52 47.12,46.89 MIC.TIP
N$28  (via drill 0.33)
  Top 0.508: v21.36,46.31 19.99,46.31 18.15,44.47 R5.2
  Bottom 0.5: 40.07,46.31 41.91,44.47 41.91,43.58 U4.29
  Bottom 0.508: v21.36,46.31 40.07,46.31
N$29  (via drill 0.33)
  Top 0.5: 18.73,36.92 R4.2
  Top 0.508: v20.45,44.98 20.45,38.13 19.22,36.9 R4.2
  Bottom 0.5: 43.18,45.25 43.18,43.58 U4.30
  Bottom 0.508: v20.45,44.98 20.45,47.52 40.91,47.52 43.18,45.25
N$31
  Top 0.5: 20.6,31.01 18.62,31.01 R2.2
  Top 0.508: 20.6,31.01 21.97,31.01 23.14,29.84 U2.10
N$35
  Top 0.5: 35.89,29.84 35.86,29.87 | D5.A 38.48,29.99
  Top 0.61: R18.2 35.89,29.84 | 35.86,29.87 D5.A
  Top 0.762: 38.48,29.99 39.39,29.99 40.22,30.82 R9.1 44.02,30.82 C19.2
PWR_IN
  Top 0.813: U6.3 7.75,42.16 10.14,42.16 D4.C D3.C 11.92,46.28 D2.C 11.92,50.44 10.92,51.45 | 10.92,51.45 D1.C | 10.92,51.45 8,51.45 C1.2
PWREN  (via drill 0.33)
  Top 0.406: U1.13 32.49,21.21 v34.78,23.5
  Bottom 0.406: U4.19 35.37,35.07 33.65,35.07 32.28,33.7 32.28,30.6 34.78,28.11 v34.78,23.5
R_AMP_OUT+  (via drill 0.33)
  Top 0.762: v50.42,54.63 42.09,54.63 U$5.7
  Bottom 0.762: JP2.5 v50.42,54.63
R_AMP_OUT-
  Bottom 0.762: JP2.9 35.69,51.58 34.16,53.11 34.16,55.65 35.94,57.43 37.32,57.43 U$5.2
RESET  (via drill 0.33)
  Top 0.406: U1.29 v33.29,8.15
  Bottom 0.406: C3.2 34.05,7.39 v33.29,8.15
  Bottom 0.5: ISP1.5 24.51,24.15 25.53,25.17 29.59,25.17 33.91,20.85 33.91,11.71
  Bottom 0.508: 33.91,11.71 33.91,11.2 34.92,10.18 R10.2 35.96,10.13 C3.2
RESET_PIN  (via drill 0.33)
  Top 0.305: U1.23 29.56,8.94 29.85,8.66 29.85,7.9 29.46,7.52 29.46,3.27 29.92,2.82 36.96,2.82 37.68,2.09 RN52_RESET.2
  Top 0.508: v50.42,28.47 50.42,3.83 48.68,2.09
  Top 0.61: RN52_RESET.2 48.68,2.09 RN52_RESET.1
  Bottom 0.406: U4.4 51.59,29.64 v50.42,28.47
ROUT+
  Bottom 0.508: U4.39 53.99,48.52 JP2.6
ROUT-
  Bottom 0.508: U4.37 51.59,45.84 JP2.10
RS  (via drill 0.33)
  Top 0.406: U1.26 30.89,7.93 v31.62,8.66 | v31.62,13.48 v35.43,13.48 | v28.32,41.93 v28.32,41.94 U3.8
  Top 0.508: 26.53,44.56 U3.8
  Top 0.61: 26.53,44.56 26.53,44.27 arc-90 R8.1
  Bottom 0.406: v31.62,8.66 v31.62,13.48 | v35.43,13.48 35.43,21.1 33.4,23.14 33.4,25.68 28.32,30.76 v28.32,41.93
RTS
  Bottom 0.305: JP1.DTR 35.17,1.17 29.22,1.17 26.92,3.47 26.92,13.41 23.28,17.06 U5.2
  Bottom 0.508: C3.1 37.96,4.72 JP1.DTR
RX  (via drill 0.33)
  Top 0.305: U1.31 34.89,5.25 JP1.RXI | v24.26,3.32 25.6,1.98 v32.16,1.98
  Bottom 0.305: U5.5 23.14,15.11 23.75,14.5 23.75,3.83 v24.26,3.32 | JP1.RXI 33.44,1.98 v32.16,1.98
RXCAN
  Top 0.5: 35.56,47.47 35.56,37.54 34.56,36.55 32.5,36.55 32.03,37.02 U2.2 | U3.4 34.66,48.37
  Top 0.508: 34.66,48.37 35.56,47.47
SCK
  Top 0.406: U1.17 27.61,13.74 25.78,15.57 25.78,20.09 ISP1.3 26.95,21.46 U2.13
STATUS_PIN  (via drill 0.33)
  Top 0.406: U1.1 46.15,8.15 49.15,11.15 v49.15,24.66
  Bottom 0.406: v49.15,24.66 53.99,29.5 U4.2
TX
  Top 0.305: U1.30 34.09,5.17 JP1.TXO
  Bottom 0.305: JP1.TXO 31.48,2.56 29.92,2.56 29.46,3.02 29.46,11.83 23.59,17.71 U5.1
TXCAN
  Top 0.5: 33.3,44.56 U2.1
  Top 0.508: 33.3,44.56 U3.1
UART_CTS
  Top 0.406: 34.16,15.31 U1.11 34.09,17.24 39.05,22.2 UART.3
  Bottom 0.406: U4.14 39.59,29.07 38.48,27.96 38.48,22.7 38.99,22.2 UART.3
UART_RTS
  Top 0.406: U1.12 33.29,19.04 38.99,24.74 UART.4
  Bottom 0.406: U4.13 40.77,30.23 UART.4
UART_RX
  Top 0.406: U1.9 35.69,15.94 36.86,17.12 UART.1
  Bottom 0.406: U4.16 37.19,29.21 36.57,28.6 36.57,19.39 38.84,17.12 UART.1
UART_TX
  Top 0.406: 34.92,15.27 U1.10 34.89,16.33 38.22,19.66 UART.2
  Bottom 0.406: U4.15 38.39,29.14 37.65,28.4 37.65,20.65 38.64,19.66 UART.2
USB+
  Bottom 0.508: U4.12 42.03,30.25 42.04,30.25 42.04,26.44 43.81,24.66 43.81,14.27 47.39,10.69 RN52_FIRMWARE.D+
USB-
  Bottom 0.508: U4.11 43.19,26.81 44.83,25.17 44.83,14.58 47.92,11.49 RN52_FIRMWARE.D-
USB_PWR  (via drill 0.33)
  Top 0.5: UPLOAD.1 6.18,13.23 10.29,13.23 10.31,13.26
  Top 0.508: 5.65,12.7 UPLOAD.1 | v20.96,15.77 18.14,12.96 C14.2 | 12.83,13.27 12.83,13.23 13.06,13.23 C15.1 C14.2 | 10.56,13.23 C11.2 10.6,13.27 v11.81,13.27 12.12,12.96 C14.2
  Top 0.61: 10.31,13.26 TXLED.A RXLED.A 11.81,23.11 11.81,40.66 15.11,43.96 D4.A
  Top 0.762: C11.2 10.29,13.23
  Bottom 0.305: v20.96,15.77 22.31,15.77 U5.4 | U5.19 12.17,11.86 11.81,12.21 11.81,12.47 | 11.81,12.47 v11.81,13.27 | U5.20 11.85,12.51 arc90 11.81,12.47
USBDM
  Bottom 0.305: U5.16 12.06,9.91
  Bottom 0.508: UPLOAD.2 10.52,12.1 12.05,10.57 C12.2 12.06,9.91
USBDP
  Bottom 0.305: C13.2 12.83,7.9 13.84,8.91 14.19,9.26 U5.15
  Bottom 0.508: UPLOAD.3 4.87,11.45 4.08,10.67 4.08,6.36 5.59,4.85 10.08,4.85 12.05,6.82 C13.2
VBUS  (via drill 0.5 pad 1.02)
  Top 0.406: 47.59,19.03 v47.62,19.07
  Top 0.762: v47.62,19.07 R11.1 47.32,30.77 C9.2 45.59,28.98 44.07,27.45 39.24,27.45 36.7,24.91 v32.13,24.91 | D3.A v17.14,46.25
  Bottom 0.508: v47.62,19.07 47.55,19.15 47.55,14.57 49.82,12.29 RN52_FIRMWARE.VBUS
  Bottom 0.762: v32.13,24.91 26.29,30.76 26.29,37.11 v17.14,46.25
XTAL1
  Top 0.406: U1.7 38.26,12.94 39.05,12.16 Y2.1
XTAL2
  Top 0.406: U1.8 38.23,13.74 39.05,14.56 Y2.3

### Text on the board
bPlace: RTS | CTS | TX | RX | UART
tNames: 12V | CANL | L- | R- | R- | L- | R+ | L+ | 3V3 | GND | L+ | R+ | CANH | EN | RX | CANL | 3V3 | GND | CANH | GND | TX | RS | RX | TX | CAN2 | CAN1 | INT0 | SCK | MOSI | MISO | CS | RST | 3V3 | GND | 3V3 | RTS | RESET | SCK | MISO | CTS | TX | GND | MOSI | 3V3 | RX | BlueSaab / v5.0 | REV | TX | RX | GND | 3V3 | DTR
bNames: 12V | CANL | L- | R- | R- | L- | R+ | L+ | GND | CANH | L+ | R+ | BT1 | BT2 | ML+ | MR+ | ML- | MR- | AGND | L- | R+ | L+ | GND | MIC BIAS | R- | GND | 3V3 | PWREN | GPIO7 | GND | GND | URX | UTX | UCTS | URTS | USB+ | USB- | GPIO9 | GPIO4 | AIC0 | GPIO2 | GPIO3 | GND | 3V3 | RESET | SCK | MISO | GND | MOSI | 3V3 | PWR | D- | VBUS | D+ | USB- | GND | USB+ | GND | TX | RX | GND | 3V3 | DTR

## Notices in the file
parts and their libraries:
SparkFun-DigitalIC: Licensing: CC v3.0 Share-Alike You are welcome to use this library for commercial purposes.
SparkFun-RF: Licensing: Creative Commons ShareAlike 4.0 International - https://creativecommons.org/licenses/by-sa/4.0
